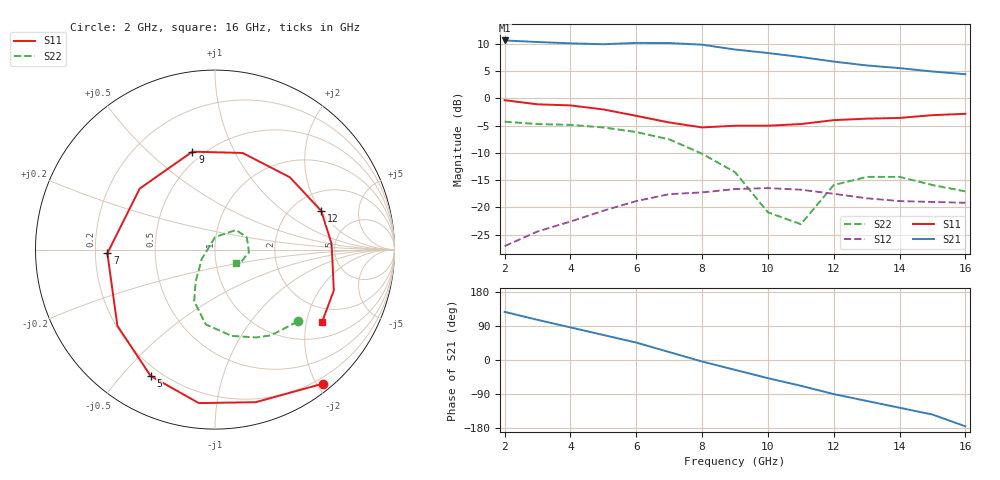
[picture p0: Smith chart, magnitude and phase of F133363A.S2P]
!ATF-13336
!S-PARAMETERS at Vds=2.5V  Id=20mA.  LAST UPDATED 07-22-92
# ghz s ma r 50
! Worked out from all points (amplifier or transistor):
!   15 points, 2 GHz to 16 GHz, reference 50 ohm
!   highest |S21| = 10.6 dB at 2 GHz (marker M1)
!   |S21| within 3 dB of that: start of sweep to 10.95 GHz
!   unconditionally stable (mu >= 1): 9.651 GHz to end of sweep
!   at 4 GHz: K = 0.54, MSG = 16.3 dB, |S12| = -22.6 dB
!   at 9 GHz: K = 0.94, MSG = 12.8 dB, |S12| = -16.7 dB
!   at 16 GHz: K = 1.42, MAG = 7.9 dB, |S12| = -19.2 dB
!   lowest NFmin = 0.70 dB at 2 GHz
!   S11 on the Smith chart (normalised r, x): 2 GHz: 0.11, -2.09; 5 GHz: 0.16, -0.60; 7 GHz: 0.25, -0.02; 9 GHz: 0.44, +0.70; 12 GHz: 2.83, +2.02; 16 GHz: 1.48, -2.48
2  0.96 -51.0  3.39 127.0  0.044 57.0  0.61 -41.0
3  0.88 -75.0  3.28 106.0  0.06 33.0  0.58 -51.0
4  0.86 -96.0  3.19 86.0  0.074 25.0  0.57 -57.0
5  0.79 -117.0  3.13 66.0  0.093 12.0  0.54 -65.0
6  0.69 -142.0  3.22 46.0  0.114 1.0  0.49 -79.0
7  0.6 -178.0  3.21 21.0  0.132 -18.0  0.42 -97.0
8  0.54 141.0  3.1 -4.0  0.137 -33.0  0.31 -112.0
9  0.56 103.0  2.8 -26.0  0.147 -48.0  0.21 -121.0
10  0.56 74.0  2.6 -48.0  0.15 -63.0  0.09 -145.0
11  0.58 44.0  2.39 -68.0  0.145 -78.0  0.07 89.0
12  0.63 20.0  2.17 -90.0  0.133 -95.0  0.16 43.0
13  0.65 3.0  2 -108.0  0.121 -107.0  0.19 21.0
14  0.66 -7.0  1.89 -126.0  0.114 -121.0  0.19 -4.0
15  0.7 -19.0  1.76 -144.0  0.112 -129.0  0.16 -28.0
16  0.72 -34.0  1.66 -175.0  0.11 -142.0  0.14 -32.0
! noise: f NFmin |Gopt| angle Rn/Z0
2  0.7  0.8  42  0.43
4  0.8  0.63  93  0.29
6  1.1  0.47  138  0.1
8  1.2  0.4  -153  0.2
10  1.3  0.47  -96  0.5
12  1.4  0.52  -45  0.88
14  1.6  0.57  -2  1.3
